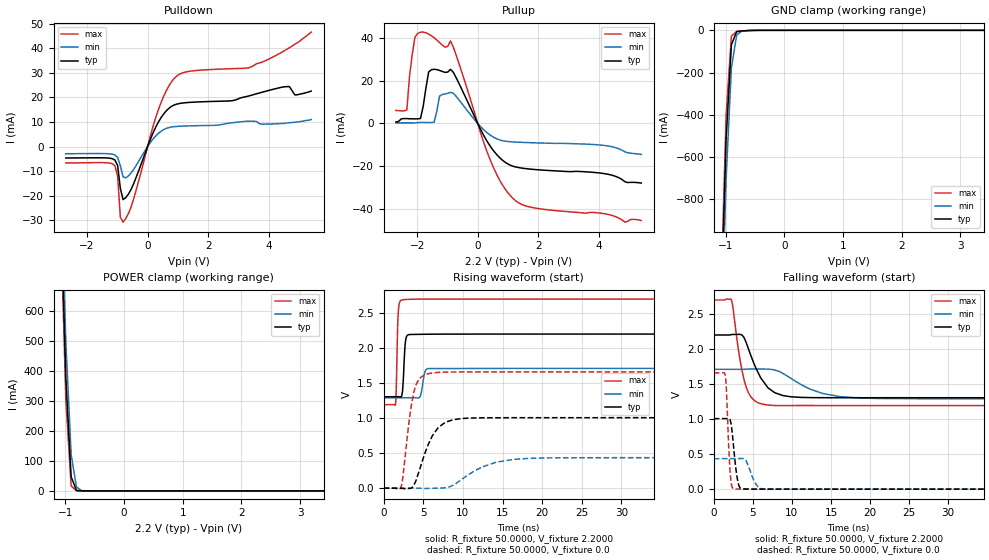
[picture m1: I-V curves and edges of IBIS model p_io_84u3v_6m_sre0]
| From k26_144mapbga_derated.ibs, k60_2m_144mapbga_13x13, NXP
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[Model] p_io_84u3v_6m_sre0
|   Model p_io_84u3v_6m_sre0
| Library cells for typ/min/max conditions are connected as defined below:
|  pad - External Pad
|  ipp_do - Core Input
|  ipp_obe - Output Buffer Enable
|  esd_boost - vdd_s_3v
|  esd_bus - vdd_s_3v
|  ipp_ina40a_3v - NC
|  ipp_ina40b_3v - NC
|  ipp_ina_3v - NC
|  ipp_ind - NC
|  ipp_ind_3v - NC
|  vdd_s_3v - vdd_s_3v
|  vdd_s_lv - vdd_s_lv
|  vss_bulk - vss_bulk
|  vss_s_lv - vss_s_lv
| All other pins connected to ground
Model_type I/O
Polarity   Non-Inverting
Enable   Active-High
Vinl =   0.6600V
Vinh =   1.6500V
Vmeas =  1.1000V
Cref =   25.0000pF
Rref =   50.0000
Vref =   0.0V
C_comp   2.2801pF   2.0930pF   2.5126pF
[Temperature Range]   25.0000   0.1250k   -40.0000
[Voltage Range]   2.2000V   1.7100V   2.7000V
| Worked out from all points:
|   slope of the pulldown table from 0 to 0.33 V, typ, clamps not added: 35.3 ohm
|   slope of the pullup table from 0 to 0.33 V, typ, clamps not added: 37.5 ohm
|   GND clamp passes 1 mA (typ) near -0.60 V on its own axis
|   POWER clamp passes 1 mA (typ) near -0.77 V on its own axis
|   rising waveform, R_fixture 50.0000, V_fixture 2.2000: 20-80 % time 250ps typ, 367ps min, 189ps max; typ from 1.3 V to 2.2 V
|   rising waveform, R_fixture 50.0000, V_fixture 0.0: 20-80 % time 2.15ns typ, 4.24ns min, 1.13ns max; typ from 0 V to 1.01 V
|   falling waveform, R_fixture 50.0000, V_fixture 2.2000: 20-80 % time 2.31ns typ, 4.46ns min, 1.38ns max; typ from 2.2 V to 1.3 V
|   falling waveform, R_fixture 50.0000, V_fixture 0.0: 20-80 % time 572ps typ, 935ps min, 382ps max; typ from 1.01 V to 0 V
[Pulldown]
|Voltage   I(typ)   I(min)   I(max)
-2.7V     -4.67mA    -2.93mA    -6.69mA
-1.08V    -5.482mA   -3.411mA   -7.784mA
-990mV    -7.73mA    -4.407mA   -11.96mA
-900mV    -17mA      -7.855mA   -28.73mA
-810mV    -21.6mA    -12.32mA   -30.8mA
-540mV    -17.32mA   -10.67mA   -24.41mA
360mV     10.04mA    5.403mA    15.15mA
900mV     17.03mA    8.127mA    28.01mA
3.33V     20.57mA    10.32mA    32.05mA
4.59V     24.4mA     9.6mA      39.55mA
4.86V     21mA       9.9mA      41.7mA
5.4V      22.6mA     11mA       46.6mA
[Pullup]
|Voltage   I(typ)   I(min)   I(max)
-2.7V     700uA      300uA      6.1mA
-2.34V    2.3mA      300uA      6.3mA
-2.16V    2.2mA      300uA      32.5mA
-1.98V    2.17mA     430uA      42.14mA
-1.89V    2.33mA     520uA      42.72mA
-1.62V    24.11mA    450uA      41.85mA
-1.44V    25.36mA    620uA      40.11mA
-1.26V    24.83mA    12.78mA    37.85mA
-900mV    25.32mA    14.58mA    38.6mA
360mV     -9.483mA   -4.889mA   -15.19mA
1.17V     -20.02mA   -8.615mA   -35.14mA
5.4V      -27.85mA   -14.46mA   -45.39mA
[GND_clamp]
|Voltage   I(typ)   I(min)   I(max)
-2.7V     -22.06A    -21.95A    -22.16A
-1.08V    -1.367A    -1.534A    -1.279A
-990mV    -516.1mA   -705.4mA   -403.6mA
-900mV    -68.3mA    -177.8mA   -27.24mA
-810mV    -6.453mA   -22.51mA   -5.196mA
-720mV    -2.652mA   -3.714mA   -3.053mA
-450mV    -86.98uA   -164.9uA   -52.14uA
5.4V      0A         0A         0A
[POWER_clamp]
|Voltage   I(typ)   I(min)   I(max)
-2.7V     15.08A     14.99A     15.18A
-1.08V    969.6mA    1.072A     917.9mA
-990mV    374.4mA    496mA      302.2mA
-900mV    47.23mA    122mA      16.99mA
-810mV    1.773mA    12.96mA    214.5uA
-720mV    53.91uA    987.1uA    2.438uA
-630mV    1.624uA    71.95uA    27.87nA
5.4V      0A         0A         0A
[Ramp]
| variable   typ   min   max
dV/dt_r  0.6037/2.1492n   0.2610/4.2402n   0.9957/1.1326n
dV/dt_f  0.5371/2.3101n   0.2515/4.4658n   0.9044/1.3766n
R_load = 50.0000
[Rising Waveform]
R_fixture= 50.0000
V_fixture= 2.2000
V_fixture_min= 1.7100
V_fixture_max= 2.7000
|time   V(typ)   V(min)   V(max)
0s        1.305V     1.291V     1.193V
1.5ns     1.305V     1.291V     1.201V
1.845ns   1.306V     1.291V     2.513V
2.29ns    1.328V     1.291V     2.686V
2.772ns   2.111V     1.291V     2.694V
3.152ns   2.192V     1.291V     2.696V
4.533ns   2.196V     1.294V     2.699V
5.165ns   2.197V     1.644V     2.7V
5.69ns    2.198V     1.708V     2.7V
50ns      2.2V       1.71V      2.7V
[Rising Waveform]
R_fixture= 50.0000
V_fixture= 0.0
V_fixture_min= 0.0
V_fixture_max= 0.0
|time   V(typ)   V(min)   V(max)
0s        1.241nV    38.83nV    72.9pV
2.202ns   -41.09uV   25.23nV    18.11mV
3.291ns   -3.38mV    -5.91uV    1.026V
3.804ns   39.87mV    -281.1nV   1.37V
4.402ns   216.9mV    -112uV     1.547V
5.683ns   637mV      -1.978mV   1.636V
6.892ns   866.1mV    -1.016mV   1.653V
9.739ns   993mV      115.9mV    1.66V
16.41ns   1.006V     411.3mV    1.659V
50ns      1.006V     435.1mV    1.659V
[Falling Waveform]
R_fixture= 50.0000
V_fixture= 2.2000
V_fixture_min= 1.7100
V_fixture_max= 2.7000
|time   V(typ)   V(min)   V(max)
0s        2.2V       1.71V      2.7V
2.234ns   2.205V     1.71V      2.706V
3.289ns   2.209V     1.71V      1.894V
3.914ns   2.153V     1.711V     1.544V
4.713ns   1.917V     1.714V     1.323V
6.243ns   1.552V     1.714V     1.213V
8.809ns   1.337V     1.653V     1.193V
12.32ns   1.307V     1.427V     1.194V
16.15ns   1.305V     1.321V     1.193V
50ns      1.305V     1.291V     1.193V
[Falling Waveform]
R_fixture= 50.0000
V_fixture= 0.0
V_fixture_min= 0.0
V_fixture_max= 0.0
|time   V(typ)   V(min)   V(max)
0s        1.006V     435.1mV    1.659V
1.465ns   1.006V     434.9mV    1.629V
1.593ns   1.007V     434.8mV    1.473V
1.887ns   1.008V     434.7mV    656.7mV
2.103ns   987.3mV    434.7mV    220.2mV
2.548ns   585.4mV    434.8mV    5.733mV
3.139ns   78.09mV    436mV      1.273mV
3.745ns   4.135mV    436mV      713.9uV
6.32ns    372uV      3.623mV    24.79uV
50ns      5.449nV    42.37nV    7.876nV
